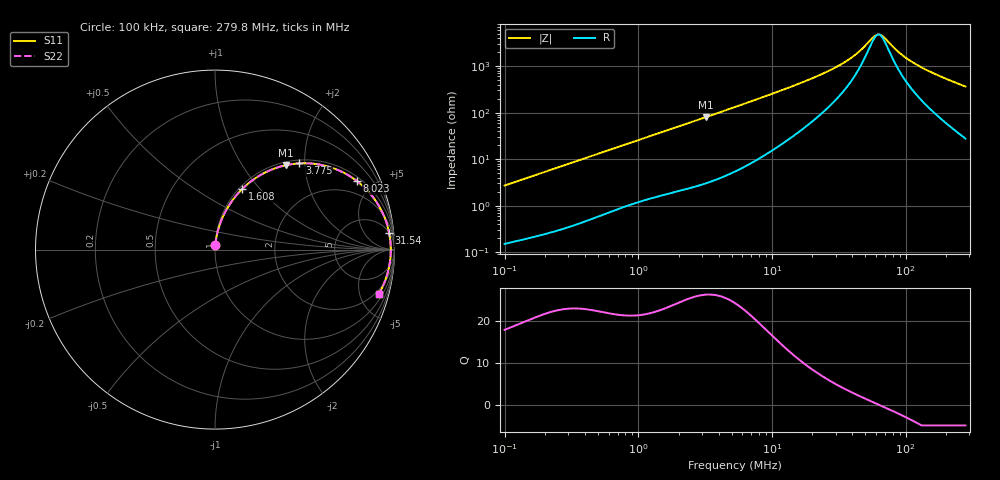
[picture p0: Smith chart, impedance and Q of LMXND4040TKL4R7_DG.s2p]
! LMXND4040TKL4R7_DG  S-PARAMETER MODEL  ( General Type )
! Model Generated by TAIYO YUDEN Corporation (http://www.ty-top.com)
! Version 1.0
! TAIYO YUDEN Control No. 191023NI43SB-FBB
! Copyright(c) 2019 TAIYO YUDEN CO.,LTD. All Rights Reserved.
! Product Description (link to TY-COMPAS)
! https://ds.yuden.co.jp/TYCOMPAS/or/detail?pn=LMXND4040TKL4R7MDG&u=M
! Products Name : Inductors
! Characteristics :
!  Inductance : 4.7 uH , SRF(min) : 35 MHz , DC Resistance(max) : 0.084 Ohm
!  Rated Current : Saturation :2000 mA , Temp Rise : 1700 mA
!  Case Size : 4.0 x 4.0 / 0.157 x 0.157 [mm/inch] , Thickness : 1.8 / 0.071 [mm/inch]
!  (Conditions: Temperature = 25 degC , DC Bias Current/Voltage = 0A / 0V)
! External Node Assignments :
!  1  o---GGG---o  2
! GND o---------o GND
! Frequency Range : 0.1MHz  -  279.750408MHz  [ 402 STEP ]
# MHz S RI R 50
! Freq[MHz].  S11 Real  S11 Imag  S21 Real  S21 Imag  S12 Real  S12 Imag  S22 Real  S22 Imag
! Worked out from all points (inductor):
!   401 points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, 100 kHz to 279.8 MHz, reference 50 ohm
!   read as one part in series: L = 4.27 uH near 104 kHz
!   highest Q = 26.4 at 3.221 MHz (marker M1), where L = 3.96 uH
!   self-resonance near 62.68 MHz
!   S11 on the Smith chart (normalised r, x): 100 kHz: 1.00, +0.05; 1.608 MHz: 1.03, +0.81; 3.775 MHz: 1.07, +1.88; 8.023 MHz: 1.21, +4.02; 31.54 MHz: 5, +20; 279.8 MHz: 1.55, -7.26
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0.1  0.00223 0.0269  0.9978 -0.0269  0.9978 -0.0269  0.00223 0.0269
0.377863  0.0139 0.0974  0.9861 -0.0974  0.9861 -0.0974  0.0139 0.0974
0.819208  0.051 0.1978  0.949 -0.1978  0.949 -0.1978  0.051 0.1978
1.427803  0.1256 0.31  0.8744 -0.31  0.8744 -0.31  0.1256 0.31
1.60831  0.1513 0.3374  0.8487 -0.3374  0.8487 -0.3374  0.1513 0.3374
2.2535  0.2493 0.4132  0.7507 -0.4132  0.7507 -0.4132  0.2493 0.4132
3.220788  0.3952 0.4703  0.6048 -0.4703  0.6048 -0.4703  0.3952 0.4703
3.774832  0.4699 0.4804  0.5301 -0.4804  0.5301 -0.4804  0.4699 0.4804
5.289144  0.6295 0.4628  0.3705 -0.4628  0.3705 -0.4628  0.6295 0.4628
8.023075  0.7904 0.3822  0.2096 -0.3822  0.2096 -0.3822  0.7904 0.3822
12.17016  0.8905 0.2786  0.1095 -0.2786  0.1095 -0.2786  0.8905 0.2786
19.9857  0.9488 0.169  0.0512 -0.169  0.0512 -0.169  0.9488 0.169
31.54342  0.9708 0.0911  0.0292 -0.0911  0.0292 -0.0911  0.9708 0.0911
42.47787  0.9769 0.0493  0.0231 -0.0493  0.0231 -0.0493  0.9769 0.0493
57.20271  0.9794 0.0114  0.0206 -0.0114  0.0206 -0.0114  0.9794 0.0114
60.711  0.9795 0.00396  0.0205 -0.00396  0.0205 -0.00396  0.9795 0.00396
65.72568  0.9795 -0.00588  0.0205 0.00588  0.0205 0.00588  0.9795 -0.00588
75.51853  0.979 -0.0232  0.021 0.0232  0.021 0.0232  0.979 -0.0232
93.93766  0.9769 -0.0514  0.0231 0.0514  0.0231 0.0514  0.9769 -0.0514
124.0157  0.9711 -0.0905  0.0289 0.0905  0.0289 0.0905  0.9711 -0.0905
180.8  0.9549 -0.1533  0.0451 0.1533  0.0451 0.1533  0.9549 -0.1533
279.7504  0.9138 -0.2451  0.0862 0.2451  0.0862 0.2451  0.9138 -0.2451
